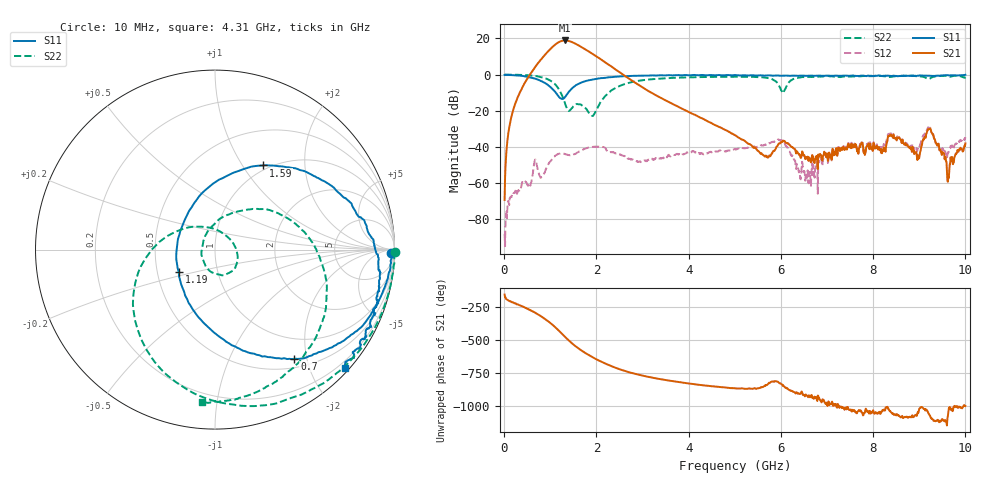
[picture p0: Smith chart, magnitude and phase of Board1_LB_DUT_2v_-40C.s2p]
! Created Tue May 27 16:01:43 2025
# hz S ma R 50
! 2 Port Network Data from SP1.SP block
! freq  magS11  angS11  magS21  angS21  magS12  angS12  magS22  angS22
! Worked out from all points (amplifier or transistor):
!   1000 points, 10 MHz to 10 GHz, reference 50 ohm
!   highest |S21| = 18.9 dB at 1.31 GHz (marker M1)
!   |S21| within 3 dB of that: 1.072 GHz to 1.632 GHz (559.9 MHz wide, 41.4 % of centre)
!   unconditionally stable (mu >= 1): 19.71 MHz to 23.9 MHz; 56.22 MHz to 65.48 MHz; 86.8 MHz to end of sweep
!   at 1.67 GHz: K = 6.72, MAG = 17.4 dB, |S12| = -41.9 dB
!   at 5.01 GHz: K = 29.14, MAG = -13.8 dB, |S12| = -41.2 dB
!   at 10 GHz: K = 10.37, MAG = -14.9 dB, |S12| = -34.5 dB
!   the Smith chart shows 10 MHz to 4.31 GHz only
!   S11 on the Smith chart (normalised r, x): 10 MHz: 58, -59; 700 MHz: 0.64, -1.79; 1.19 GHz: 0.65, -0.17; 1.59 GHz: 0.94, +1.24; 4.31 GHz: 0.09, -2.58
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1e7  0.9832 -1.0  0.0003449 -153.6  3.966e-05 102.1  1.005 -0.8
1.9e8  0.9676 -12.9  0.09924 147.9  0.0004647 87.9  0.9951 -17.1
7e8  0.7514 -54.0  1.809 61.9  0.003538 65.1  0.9118 -72.0
9.4e8  0.529 -81.4  4.246 6.5  0.003014 113.7  0.751 -110.4
1.08e9  0.3642 -108.3  6.373 -33.9  0.00531 97.1  0.5794 -141.0
1.19e9  0.238 -147.9  7.982 -70.2  0.006448 77.5  0.3874 -173.3
1.25e9  0.2128 177.3  8.569 -91.5  0.00665 68.8  0.2759 164.1
1.31e9  0.231 139.0  8.815 -112.8  0.006417 60.8  0.1759 133.3
1.44e9  0.3791 89.1  8.238 -156.2  0.005915 57.6  0.1081 18.2
1.59e9  0.5402 60.3  6.69 161.1  0.007065 59.2  0.1535 -51.0
1.68e9  0.6085 48.9  5.745 138.8  0.008155 53.7  0.1429 -78.5
1.9e9  0.728 30.5  3.867 91.7  0.01 32.2  0.07392 -176.9
2.12e9  0.8022 18.0  2.539 51.7  0.01005 7.2  0.1964 73.3
2.54e9  0.895 -0.3  1.083 -7.7  0.006029 -10.9  0.5095 10.7
3.34e9  0.9524 -21.6  0.2488 -75.8  0.004664 11.3  0.7717 -50.3
4.31e9  0.9769 -42.4  0.06041 -125.8  0.00633 -2.6  0.8534 -95.0
5.01e9  0.9762 -56.0  0.0211 -148.3  0.008699 -8.7  0.8754 -119.5
6.67e9  0.9399 -87.9  0.005268 159.5  0.002691 165.1  0.8666 -150.6
8.34e9  0.9299 -133.1  0.01981 50.2  0.02251 55.2  0.8615 167.5
9.23e9  0.9326 -157.2  0.03129 5.3  0.03361 12.6  0.7783 161.7
9.62e9  0.9603 -167.6  0.001095 0.2  0.006475 50.2  0.9002 152.7
1e10  0.9921 -179.5  0.01253 76.7  0.01875 68.8  0.8461 144.6
